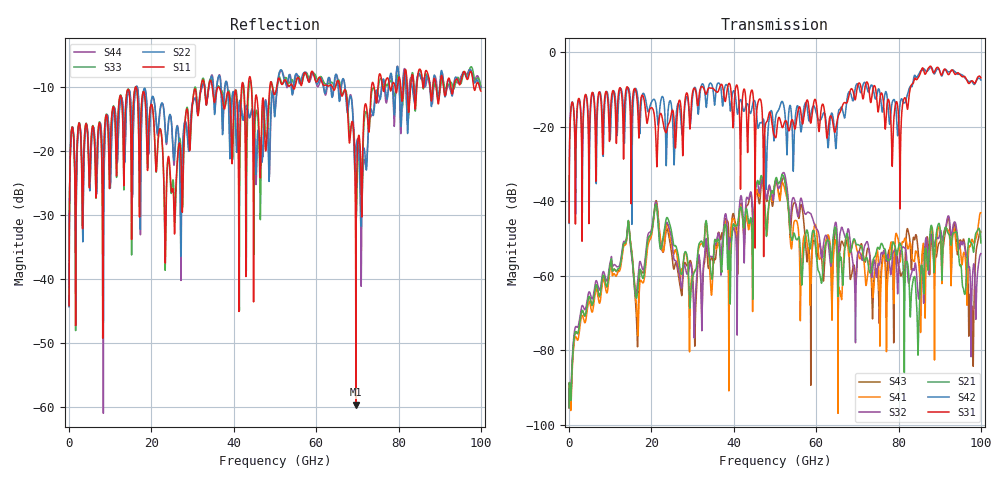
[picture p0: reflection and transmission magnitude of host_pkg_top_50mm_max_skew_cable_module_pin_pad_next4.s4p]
# Hz S RI R 50
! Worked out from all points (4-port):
!   10000 points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, 10 MHz to 100 GHz, reference 50 ohm
!   strongest paths, dB at 10 MHz, 25.01 GHz, 50.01 GHz, 75.01 GHz, 100 GHz:
!     S31: -45.7, -15.7, -22.8, -16.0, -6.9
!     S42: -45.9, -16.0, -18.9, -10.1, -7.5
!     S21: -95.4, -49.0, -34.7, -52.4, -51.2
!     S32: -95.4, -51.0, -35.4, -57.0, -54.0
!     S41: -95.3, -52.8, -34.9, -54.4, -43.1
!     S43: -95.4, -54.9, -35.3, -60.8, -48.2
!   lowest |S11| = -59.7 dB at 69.63 GHz (marker M1), VSWR 1.00, Z = 50.1 - j0.0805 ohm
!   |S11| at or under -10 dB: start of sweep to 32.06 GHz; 34.75 GHz to 41.92 GHz (7.172 GHz wide, 18.7 % of centre); 65.74 GHz to 73.45 GHz (7.708 GHz wide, 11.1 % of centre)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
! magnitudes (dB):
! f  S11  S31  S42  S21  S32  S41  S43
! 10 MHz  -44.2  -45.7  -45.9  -95.4  -95.4  -95.3  -95.4
! 52.05 GHz  -9.3  -19.7  -13.9  -33.3  -32.3  -35.5  -33.8
! 69.63 GHz  -59.7  -12.1  -9.0  -51.3  -67.6  -51.8  -61.7
! 84.72 GHz  -8.1  -7.0  -6.3  -81.0  -65.1  -55.2  -52.8
! 91.98 GHz  -9.0  -5.9  -5.2  -48.5  -44.1  -47.7  -44.6
! 97.88 GHz  -8.3  -7.7  -8.0  -51.7  -62.4  -50.2  -68.8
! 100 GHz  -10.7  -6.9  -7.5  -51.2  -54.0  -43.1  -48.2
